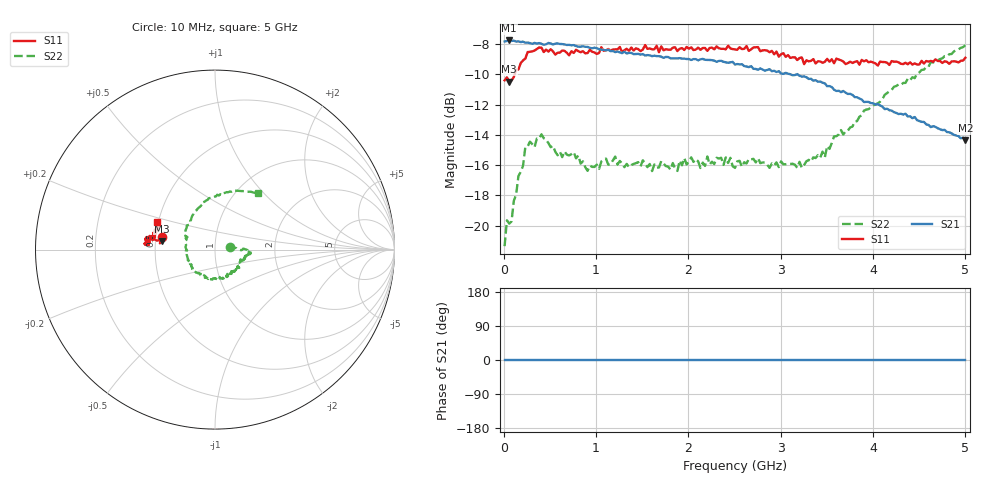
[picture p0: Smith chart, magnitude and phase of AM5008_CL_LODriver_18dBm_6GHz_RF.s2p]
!Keysight Technologies,N5245B,MY58422270,A.16.20.02
!Mixer S2P File: Scalar Mixer Measurement
!Calibration State: On
!Parameters: Stimulus Freq, S11, SC21, SC12, S22
# Hz  S  DB  R  50.0
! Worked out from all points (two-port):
!   201 points, 10 MHz to 5 GHz, reference 50 ohm
!   highest |S21| = -7.76 dB at 59.9 MHz (marker M1); lowest = -14.4 dB at 5 GHz (marker M2)
!   |S21| within 3 dB of the highest: start of sweep to 3.5 GHz
!   lowest |S11| = -10.5 dB at 59.9 MHz (marker M3), VSWR 1.85, Z = 27.1 + j2.85 ohm
!   |S11| at or under -10 dB: start of sweep to 118.7 MHz
!   |S22| runs from -21.4 to -8.1 dB; largest |S21 - S12| = 0.41
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1e7  -10.40 166.0  -7.83 0.0  -200.00 90.0  -21.36 11.0
3.495e7  -10.20 173.5  -7.80 0.0  -200.00 90.0  -19.65 3.8
5.99e7  -10.49 170.8  -7.76 0.0  -200.00 90.0  -19.87 2.9
2.3455e8  -8.96 170.9  -7.91 0.0  -200.00 90.0  -14.80 -0.9
2.8445e8  -8.51 171.4  -7.94 0.0  -200.00 90.0  -14.45 -3.2
4.092e8  -8.24 171.8  -7.98 0.0  -200.00 90.0  -13.96 -4.9
5.8385e8  -8.57 173.4  -7.95 0.0  -200.00 90.0  -15.35 -12.3
8.583e8  -8.47 175.2  -8.14 0.0  -200.00 90.0  -15.75 -19.8
1.68165e9  -8.54 174.3  -8.80 0.0  -200.00 90.0  -16.16 -53.0
1.88125e9  -8.46 174.3  -8.95 0.0  -200.00 90.0  -16.39 -63.3
2.03095e9  -8.21 174.0  -9.05 0.0  -200.00 90.0  -15.49 -74.4
2.13075e9  -8.37 172.7  -9.01 0.0  -200.00 90.0  -16.19 -80.3
2.2056e9  -8.45 172.4  -9.05 0.0  -200.00 90.0  -15.43 -85.4
2.505e9  -8.35 171.9  -9.35 0.0  -200.00 90.0  -16.19 -115.3
2.7545e9  -8.20 170.2  -9.69 0.0  -200.00 90.0  -15.55 -140.0
3.17865e9  -9.06 167.9  -9.98 0.0  -200.00 90.0  -16.18 -173.4
3.3533e9  -8.99 166.9  -10.42 0.0  -200.00 90.0  -15.49 167.6
3.47805e9  -9.17 166.6  -10.60 0.0  -200.00 90.0  -15.48 155.7
3.6527e9  -9.07 164.5  -11.17 0.0  -200.00 90.0  -13.68 139.3
4.17665e9  -9.38 159.9  -12.37 0.0  -200.00 90.0  -11.11 100.2
4.62575e9  -9.11 155.9  -13.49 0.0  -200.00 90.0  -9.18 72.5
5e9  -8.90 154.2  -14.37 0.0  -200.00 90.0  -8.07 52.5
